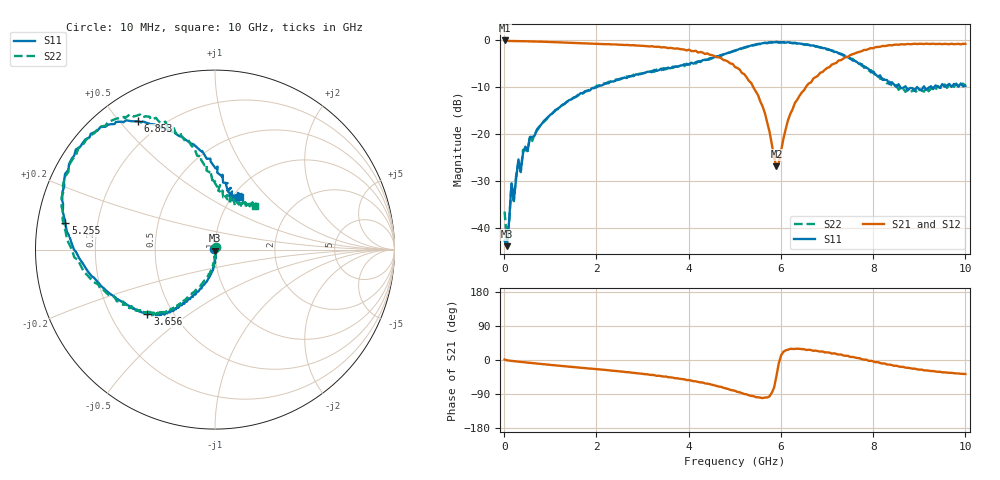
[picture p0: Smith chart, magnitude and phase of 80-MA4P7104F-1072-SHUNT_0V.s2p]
!Agilent Technologies,E8364C,MY48140145,A.09.42.15
!Agilent E8364C: A.09.42.15
!Date: Wednesday, December 02, 2020 11:05:53
!Correction: S11(Full 2 Port(1,2))
!S21(Full 2 Port(1,2))
!S12(Full 2 Port(1,2))
!S22(Full 2 Port(1,2))
!S2P File: Measurements: S11, S21, S12, S22:
# Hz S  dB  R 50
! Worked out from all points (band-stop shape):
!   201 points, 10 MHz to 10 GHz, reference 50 ohm
!   highest |S21| = -0.10 dB at 10 MHz (marker M1); lowest = -26.9 dB at 5.904 GHz (marker M2)
!   |S21| within 3 dB of the highest: start of sweep to 4.449 GHz; 7.535 GHz to end of sweep
!   lowest |S11| = -43.9 dB at 59.95 MHz (marker M3), VSWR 1.01, Z = 50.1 - j0.634 ohm
!   |S11| at or under -10 dB: start of sweep to 2.016 GHz; 8.585 GHz to 8.68 GHz (95.09 MHz wide, 1.1 % of centre); 8.709 GHz to 9.093 GHz (383.6 MHz wide, 4.31 % of centre)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
!   |S22| runs from -42.9 to -0.5 dB; largest |S21 - S12| = 0.041
!   S11 on the Smith chart (normalised r, x): 10 MHz: 0.99, +0.00; 3.656 GHz: 0.36, -0.35; 5.255 GHz: 0.08, +0.09; 6.853 GHz: 0.12, +0.56; 10 GHz: 1.08, +0.71
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1e7  -42.74 169.6  -0.10 1.3  -0.15 -1.1  -36.52 71.7
5.995e7  -43.91 -83.7  -0.20 -0.9  -0.19 -1.1  -42.88 -98.8
1.5985e8  -30.53 -84.5  -0.22 -2.5  -0.22 -2.5  -30.64 -83.5
2.098e8  -34.14 -82.4  -0.22 -3.1  -0.22 -3.2  -34.34 -92.7
3.097e8  -25.44 -89.7  -0.25 -4.3  -0.26 -4.5  -25.94 -88.3
3.5965e8  -28.04 -82.1  -0.26 -5.1  -0.24 -5.1  -28.14 -94.4
4.096e8  -24.05 -92.1  -0.27 -5.6  -0.27 -5.7  -23.38 -91.6
5.095e8  -23.59 -89.4  -0.28 -6.9  -0.28 -7.0  -23.67 -97.0
5.5945e8  -20.64 -94.9  -0.31 -7.6  -0.32 -7.6  -20.41 -95.0
1.7083e9  -11.41 -114.1  -0.68 -21.0  -0.67 -20.8  -11.25 -117.7
3.35665e9  -6.43 -131.2  -1.44 -41.5  -1.46 -42.2  -6.42 -131.5
3.65635e9  -5.67 -136.4  -1.77 -46.4  -1.72 -47.1  -5.97 -136.4
5.005e9  -2.22 -179.0  -5.76 -81.3  -5.65 -81.2  -2.32 -175.7
5.25475e9  -1.44 170.0  -7.92 -90.4  -7.87 -90.9  -1.53 173.1
5.65435e9  -0.58 153.2  -15.63 -99.1  -15.56 -99.2  -0.64 154.2
5.9041e9  -0.40 144.3  -26.93 -41.8  -26.91 -41.7  -0.47 143.7
6.3037e9  -0.59 133.1  -13.41 29.2  -13.37 30.1  -0.66 130.2
6.7033e9  -1.17 124.5  -8.22 24.3  -8.18 25.9  -1.25 120.8
6.85315e9  -1.59 120.9  -6.99 22.3  -6.94 23.4  -1.55 117.4
8.35165e9  -9.43 77.9  -1.09 -12.1  -1.18 -12.7  -8.86 85.5
8.95105e9  -10.01 68.2  -0.87 -24.5  -0.76 -24.1  -11.34 66.0
1e10  -9.77 64.6  -0.83 -37.0  -0.84 -37.2  -9.67 47.4
